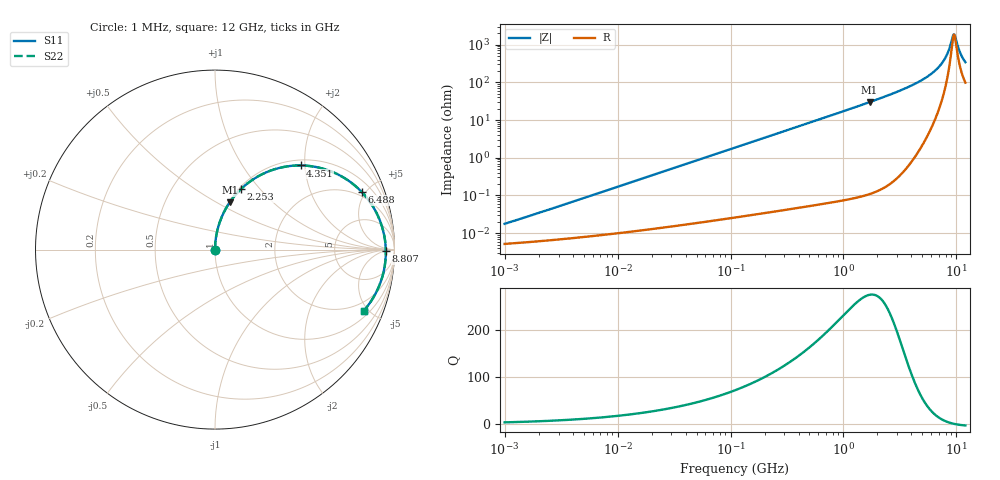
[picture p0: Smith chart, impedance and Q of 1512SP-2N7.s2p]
# MHz  S  MA  R  50
!Freq  MagS11  AngS11  MagS21  AngS21  MagS12  AngS12  MagS22  AngS22
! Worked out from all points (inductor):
!   801 points, 1 MHz to 12 GHz, reference 50 ohm
!   read as one part in series: L = 2.7 nH near 1.048 MHz
!   highest Q = 274 at 1.7 GHz (marker M1), where L = 2.79 nH
!   self-resonance near 9.542 GHz
!   S11 on the Smith chart (normalised r, x): 1 MHz: 1.00, +0.00; 2.253 GHz: 1.02, +0.79; 4.351 GHz: 1.12, +1.90; 6.488 GHz: 1.67, +4.69; 8.807 GHz: 40, -6; 12 GHz: 1.35, -4.69
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1  0.000172 72.4  0.9999 -0.0  0.9999 -0.0  0.000172 72.4
4.828773  0.0007956 84.3  0.9999 -0.0  0.9999 -0.0  0.0007956 84.3
23.04466  0.003781 87.7  0.9999 -0.2  0.9999 -0.2  0.003781 87.7
109.9775  0.01803 88.1  0.9996 -1.1  0.9996 -1.1  0.01803 88.1
524.8526  0.08598 84.4  0.9958 -5.3  0.9958 -5.3  0.08597 84.4
978.3857  0.16 79.9  0.9864 -9.8  0.9864 -9.8  0.16 79.9
1699.665  0.2767 72.6  0.9599 -17.2  0.9599 -17.2  0.2767 72.6
2253.417  0.3648 66.9  0.9297 -22.8  0.9297 -22.8  0.3647 66.9
2534.394  0.4087 64.0  0.9109 -25.8  0.9109 -25.8  0.4086 64.0
3360.101  0.5331 55.3  0.8426 -34.4  0.8426 -34.4  0.533 55.3
4351.351  0.6688 44.5  0.7353 -44.8  0.7353 -44.8  0.6687 44.5
5376.291  0.7857 33.3  0.5996 -55.2  0.5996 -55.2  0.7856 33.3
6488.36  0.8779 21.5  0.4348 -65.5  0.4348 -65.5  0.8778 21.5
7212.142  0.9171 14.2  0.325 -70.7  0.325 -70.7  0.917 14.2
7830.456  0.9382 8.2  0.2338 -73.2  0.2338 -73.2  0.9382 8.2
8304.306  0.9476 3.9  0.1675 -72.6  0.1675 -72.6  0.9475 3.9
8806.831  0.9518 -0.4  0.1035 -65.4  0.1035 -65.4  0.9518 -0.4
9230.659  0.9514 -3.9  0.06139 -42.8  0.06139 -42.8  0.9515 -3.9
9450.161  0.9501 -5.6  0.05107 -18.2  0.05107 -18.2  0.9501 -5.6
9674.883  0.9479 -7.3  0.05439 9.9  0.05439 9.9  0.9479 -7.3
10881.24  0.9261 -15.7  0.1599 51.1  0.1599 51.1  0.9262 -15.7
12000  0.8964 -22.3  0.257 51.2  0.257 51.2  0.8966 -22.3
